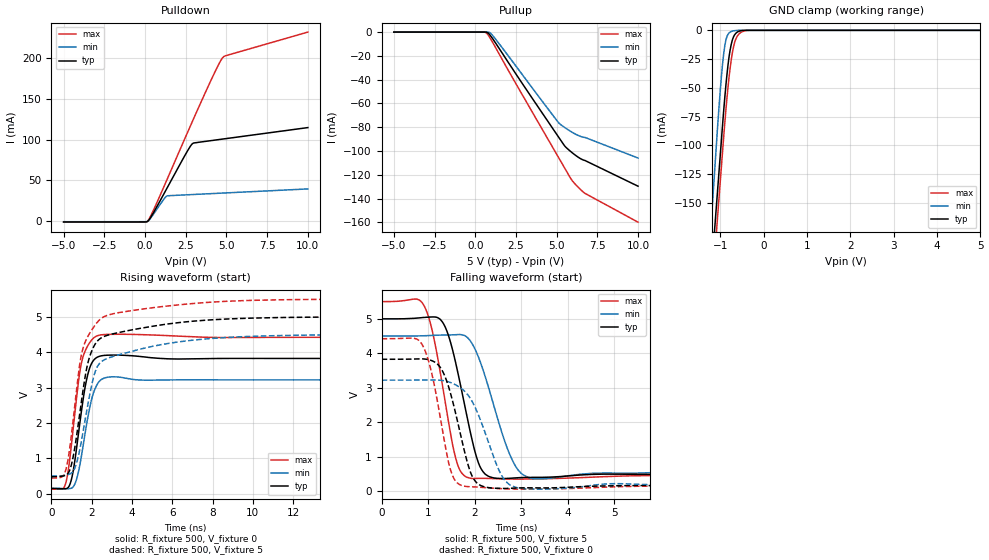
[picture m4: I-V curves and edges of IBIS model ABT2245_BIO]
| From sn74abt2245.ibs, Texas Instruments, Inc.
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[Model]   ABT2245_BIO
Model_type  I/O
Vinl=0.8
Vinh=2.0
Enable   Active-Low
Vref =   0
Rref =   500
Cref =   50p
Vmeas =   1.5
| variable   typ   min   max
C_comp   5.99pF   4.83pF   8.42pF
| C_pullup   4.00pF   1.74pF   5.45pF
| C_pulldown   3.59pF   0.08pF   7.11pF
| C_tri-state   5.99pF   4.83pF   8.42pF
[Temperature Range]   40   -40   100
| Ambient temperature   25   -40   85
[Voltage range]   5   4.5   5.5
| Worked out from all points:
|   slope of the pulldown table from 0 to 0.75 V, typ, clamps not added: 38.5 ohm
|   slope of the pullup table from 0 to 0.75 V, typ, clamps not added: 2.01 kohm
|   GND clamp passes 1 mA (typ) near -0.58 V on its own axis
|   rising waveform, R_fixture 500, V_fixture 0: 20-80 % time 548ps typ, 573ps min, 533ps max; typ from 0.152 V to 3.82 V
|   falling waveform, R_fixture 500, V_fixture 5: 20-80 % time 436ps typ, 551ps min, 394ps max; typ from 5 V to 0.483 V
|   rising waveform, R_fixture 500, V_fixture 5: 20-80 % time 865ps typ, 995ps min, 905ps max; typ from 0.483 V to 5 V
|   falling waveform, R_fixture 500, V_fixture 0: 20-80 % time 407ps typ, 527ps min, 362ps max; typ from 3.82 V to 0.152 V
[GND Clamp]
| ABT2245_BIO
|   Voltage   I(typ)   I(min)   I(max)
-5V       -2.209A    -2.394A    -2.256A
-1.235V   -224.1mA   -179.4mA   -247.8mA
-1.21V    -211.4mA   -165.2mA   -235.1mA
-1.12V    -165.9mA   -114.4mA   -189.4mA
-1.075V   -143.6mA   -89.01mA   -166.6mA
-975mV    -94.09mA   -38.95mA   -117.1mA
-900mV    -58.53mA   -13.56mA   -80.78mA
-825mV    -30.01mA   -3.417mA   -49.24mA
-750mV    -12.03mA   -1.023mA   -25.51mA
-625mV    -1.892mA   -93.96uA   -5.959mA
-400mV    -7.598uA   -3.5nA     -166.3uA
5V        82.81pA    75.18pA    1.574nA
[Pulldown]
| ABT2245_BIO
|   Voltage   I(typ)   I(min)   I(max)
-5V       -994.7uA   -709uA     -1.289mA
125mV     -620.4uA   -543uA     -496.4uA
450mV     7.995mA    6.561mA    10.56mA
1.33V     39.7mA     30.7mA     50.02mA
2.475V    81.41mA    32.16mA    102.5mA
2.88V     94.29mA    32.56mA    120.9mA
3.025V    95.86mA    32.7mA     127.4mA
4.21V     99.07mA    33.85mA    179.3mA
4.575V    100.1mA    34.2mA     194mA
4.775V    100.6mA    34.4mA     200.5mA
4.99V     101.2mA    34.61mA    202.9mA
10V       114.6mA    39.48mA    231.6mA
[Pullup]
| ABT2245_BIO
|   Voltage   I(typ)   I(min)   I(max)
-5V       -7.103pA   -6.281pA   -5.99pA
480mV     -55.47nA   -14.74pA   -4.438uA
685mV     -67.14uA   -104.3nA   -751.4uA
900mV     -2.376mA   -489.1uA   -4.672mA
1.19V     -7.945mA   -4.848mA   -11.53mA
2.395V    -33.06mA   -26.63mA   -40.89mA
5.12V     -88.31mA   -76.25mA   -105.5mA
5.525V    -96.21mA   -80.52mA   -115.1mA
5.975V    -101.7mA   -84.47mA   -125.3mA
6.43V     -106.1mA   -87.52mA   -131.9mA
6.735V    -108mA     -88.57mA   -135.6mA
10V       -129.6mA   -105.9mA   -159.9mA
[Ramp]
| ABT2245_BIO
| variable   typ   min   max
dV/dt_r   2.26/5.72E-10   1.90/6.01E-10   2.62/5.52E-10
dV/dt_f   2.82/4.57E-10   2.51/5.85E-10   3.14/4.11E-10
R_load = 500
[Rising Waveform]
| ABT2245_BIO
R_fixture =   500
C_fixture =   0
L_fixture =   0
V_fixture =   0
V_fixture_min = 0
V_fixture_max = 0
|   Time   V(typ)   V(min)   V(max)
0s        152.2mV    159.5mV    135.3mV
540ps     143.5mV    149.2mV    142.5mV
700ps     146.3mV    143.5mV    279.1mV
940ps     301.7mV    153mV      1.12V
1.16ns    926.2mV    275.7mV    2.255V
1.465ns   2.227V     983.2mV    3.624V
1.805ns   3.369V     2.152V     4.183V
2.095ns   3.772V     2.861V     4.401V
2.455ns   3.894V     3.218V     4.488V
49.99ns   3.823V     3.218V     4.419V
[Falling Waveform]
| ABT2245_BIO
R_fixture =   500
C_fixture =   0
L_fixture =   0
V_fixture =   5
V_fixture_min = 4.5
V_fixture_max = 5.5
|   Time   V(typ)   V(min)   V(max)
0s        4.999V     4.499V     5.499V
925ps     5.041V     4.508V     5.347V
1.115ns   5.054V     4.519V     4.488V
1.4ns     4.652V     4.53V      2.312V
1.645ns   3.391V     4.541V     718.6mV
1.94ns    1.504V     4.288V     362.1mV
2.215ns   500.7mV    3.367V     365.2mV
2.785ns   370.2mV    960.7mV    345.4mV
3.265ns   393.1mV    356.2mV    348mV
49.99ns   483mV      500.4mV    445.1mV
[Rising Waveform]
| ABT2245_BIO
R_fixture =   500
C_fixture =   0
L_fixture =   0
V_fixture =   5
V_fixture_min = 4.5
V_fixture_max = 5.5
|   Time   V(typ)   V(min)   V(max)
0s        482.9mV    500.3mV    445.1mV
740ps     538mV      531.4mV    732.5mV
970ps     776.7mV    579mV      1.558V
1.21ns    1.482V     803.6mV    2.743V
1.44ns    2.405V     1.345V     3.785V
1.67ns    3.292V     2.078V     4.278V
2.265ns   4.303V     3.575V     4.836V
3.35ns    4.556V     3.926V     5.117V
11.24ns   4.977V     4.468V     5.478V
49.99ns   4.999V     4.499V     5.499V
[Falling Waveform]
| ABT2245_BIO
R_fixture =   500
C_fixture =   0
L_fixture =   0
V_fixture =   0
V_fixture_min = 0
V_fixture_max = 0
|   Time   V(typ)   V(min)   V(max)
0s        3.824V     3.218V     4.421V
875ps     3.836V     3.221V     4.242V
1.055ns   3.796V     3.223V     3.542V
1.245ns   3.617V     3.216V     2.252V
1.485ns   2.813V     3.146V     592.7mV
1.85ns    791.7mV    2.796V     124.8mV
2.065ns   211.6mV    2.256V     110.9mV
2.595ns   72.52mV    409.1mV    64.75mV
3.12ns    91mV       61.72mV    51.23mV
49.99ns   152.2mV    159.5mV    135.3mV
